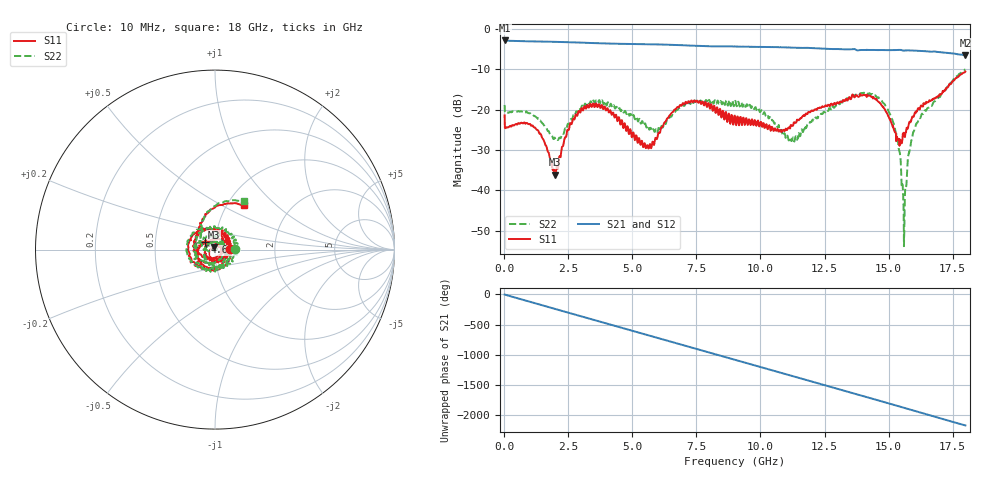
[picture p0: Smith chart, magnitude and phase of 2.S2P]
!Agilent Technologies,E5071C,MY46316741,A.11.02
!Date: Tue Sep 22 10:33:48 2020
!Data & Calibration Information:
!Freq	S11:SOLT4(ON)	S21:SOLT4(ON)	S12:SOLT4(ON)	S22:SOLT4(ON)
!PortZ  Port1:50+j0  Port2:50+j0
!Above PortZ is port z conversion or system Z0 setting when saving the data.
!When reading, reference impedance value at option line is always used.
# Hz S dB R 50
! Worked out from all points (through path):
!   1561 points, 10 MHz to 18 GHz, reference 50 ohm
!   highest |S21| = -2.91 dB at 10 MHz (marker M1); lowest = -6.6 dB at 18 GHz (marker M2)
!   group delay of S21, straight-line fit = 335 ps
!   lowest |S11| = -36.1 dB at 1.982 GHz (marker M3), VSWR 1.03, Z = 49.5 + j1.46 ohm
!   |S11| at or under -10 dB: start of sweep to end of sweep
!   |S22| runs from -53.8 to -10.1 dB; largest |S21 - S12| = 0.018
!   S11 on the Smith chart (normalised r, x): 10 MHz: 1.18, +0.01; 4.611 GHz: 0.89, +0.07; 18 GHz: 1.19, +0.65
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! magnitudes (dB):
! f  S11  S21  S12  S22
! 10 MHz  -21.4  -2.9  -2.9  -18.9
! 1.255 GHz  -24.9  -3.2  -3.2  -22.0
! 1.982 GHz  -36.1  -3.3  -3.3  -27.1
! 2.512 GHz  -25.1  -3.4  -3.4  -23.6
! 3.02 GHz  -19.6  -3.4  -3.5  -19.2
! 3.746 GHz  -19.6  -3.6  -3.6  -18.4
! 4.611 GHz  -23.4  -3.8  -3.8  -20.0
! 5.58 GHz  -28.8  -3.8  -3.9  -24.2
! 6.007 GHz  -26.0  -3.9  -3.9  -24.8
! 7.241 GHz  -18.3  -4.2  -4.2  -18.4
! 9.005 GHz  -21.8  -4.4  -4.5  -18.0
! 10.09 GHz  -23.8  -4.5  -4.5  -21.1
! 11.16 GHz  -24.6  -4.7  -4.7  -26.9
! 12.01 GHz  -20.2  -4.8  -4.8  -22.7
! 13.96 GHz  -16.6  -5.3  -5.3  -16.0
! 15 GHz  -21.7  -5.3  -5.3  -20.5
! 15.38 GHz  -27.4  -5.3  -5.4  -28.9
! 15.54 GHz  -27.3  -5.4  -5.2  -38.5
! 15.61 GHz  -26.3  -5.4  -5.3  -50.4
! 15.82 GHz  -23.0  -5.4  -5.4  -30.2
! 16.12 GHz  -20.2  -5.5  -5.5  -23.3
! 18 GHz  -10.6  -6.6  -6.6  -10.1
